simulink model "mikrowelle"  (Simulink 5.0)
settings: Solver=FixedStepDiscrete  StartTime=0.0  StopTime=100  FixedStep=0.0001  RelTol=1e-3
libraries: simulink x3

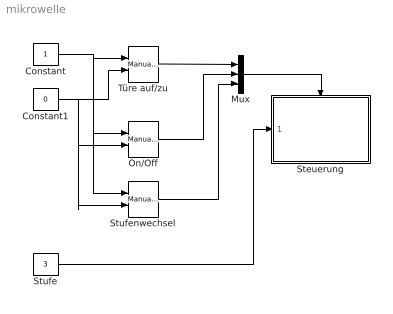
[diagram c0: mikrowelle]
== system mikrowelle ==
  Constant : Constant
  Constant1 : Constant  Value=0
  Mux : Mux  Inputs=3
  On/Off : simulink/Signal Routing/Manual Switch  sw=0  action=0
  Steuerung : Stateflow chart  TreatAsAtomicUnit=on
  Stufe : Constant  Value=3
  Stufenwechsel : simulink/Signal Routing/Manual Switch  sw=0  action=0
  Türe auf/zu : simulink/Signal Routing/Manual Switch  sw=1  action=0
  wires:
  Constant1/1 -> Türe auf/zu/2, On/Off/2, Stufenwechsel/2
  Constant/1 -> Türe auf/zu/1, On/Off/1, Stufenwechsel/1
  Mux/1 -> Steuerung/Trigger
  Türe auf/zu/1 -> Mux/1
  On/Off/1 -> Mux/2
  Stufe/1 -> Steuerung/1(stufe)
  Stufenwechsel/1 -> Mux/3

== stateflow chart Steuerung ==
  state Open
  state Closed
    state Off
    state On
      state Stufe1
      state Stufe2
      state Stufe3
      (default) -> (junction 10)
      (junction 10) -> Stufe1 : [stufe==1]
      (junction 10) -> Stufe2 : [stufe==2]
      (junction 10) -> Stufe3 : [stufe==3]
      On -> (junction 10) : change
    Off -> On : switch
    On -> Off : switch
    (default) -> Off
  Open -> Closed : door
  Closed -> Open : door
  (default) -> Open
